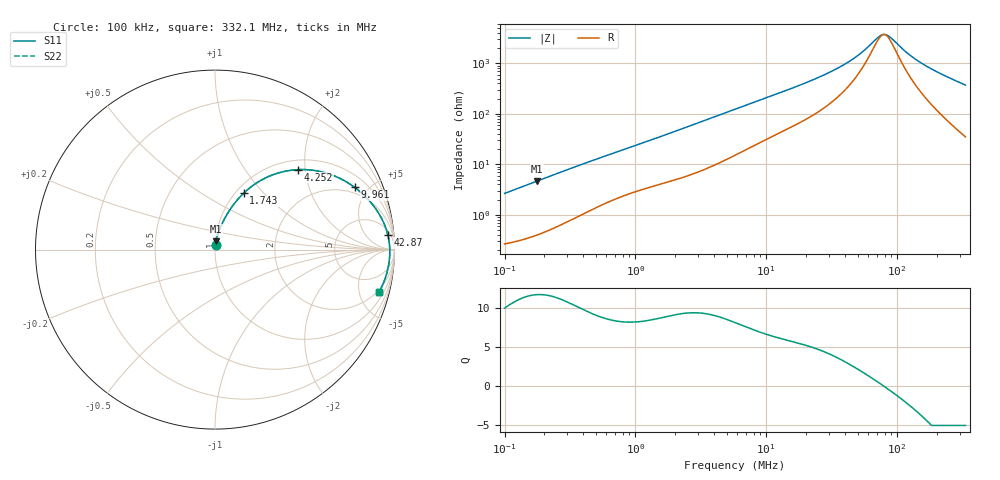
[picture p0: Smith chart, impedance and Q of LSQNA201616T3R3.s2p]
! LSQNA201616T3R3  S-PARAMETER MODEL  ( General Type )
! Model Generated by TAIYO YUDEN Corporation (http://www.ty-top.com)
! Version 2.0
! TAIYO YUDEN Control No. 100810NF25SB-FKC
! Copyright(c) 2007 TAIYO YUDEN CO.,LTD. All Rights Reserved.
! Product Description (link to TY-COMPAS)
! https://ds.yuden.co.jp/TYCOMPAS/or/detail?pn=LSQNA201616T3R3M&u=M
! Products Name : Inductors
! Characteristics :
!  Inductance : 3.3 uH , SRF(min) : 55 MHz , DC Resistance(max) : 0.26 Ohm
!  Rated Current : Saturation :400 mA , Temp Rise : 800 mA (40 degC)
!  Case Size : 2.0 x 1.6 / 0.079 x 0.063 [mm/inch] , Thickness : 1.6 / 0.063 [mm/inch]
!  (Conditions: Temperature = 25 degC , DC Bias Current/Voltage = 0A / 0V)
! External Node Assignments :
!  1  o---GGG---o  2
! GND o---------o GND
! Frequency Range : 0.1MHz  -  332.076389MHz  [ 402 STEP ]
# MHz S RI R 50
! Freq[MHz].  S11 Real  S11 Imag  S21 Real  S21 Imag  S12 Real  S12 Imag  S22 Real  S22 Imag
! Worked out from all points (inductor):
!   401 points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, 100 kHz to 332.1 MHz, reference 50 ohm
!   read as one part in series: L = 4.2 uH near 104.1 kHz
!   highest Q = 11.7 at 176.4 kHz (marker M1), where L = 4.18 uH
!   self-resonance near 79.18 MHz
!   S11 on the Smith chart (normalised r, x): 100 kHz: 1.01, +0.05; 1.743 MHz: 1.09, +0.78; 4.252 MHz: 1.21, +1.83; 9.961 MHz: 1.62, +4.09; 42.87 MHz: 8, +20; 332.1 MHz: 1.70, -7.41
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0.1  0.00334 0.0263  0.9967 -0.0263  0.9967 -0.0263  0.00334 0.0263
0.176395  0.00607 0.0459  0.9939 -0.0459  0.9939 -0.0459  0.00607 0.0459
0.388873  0.0195 0.0963  0.9805 -0.0963  0.9805 -0.0963  0.0195 0.0963
0.840088  0.06 0.1841  0.94 -0.1841  0.94 -0.1841  0.06 0.1841
1.512219  0.1326 0.2862  0.8674 -0.2862  0.8674 -0.2862  0.1326 0.2862
1.742755  0.1603 0.3149  0.8397 -0.3149  0.8397 -0.3149  0.1603 0.3149
2.613956  0.2717 0.3945  0.7283 -0.3945  0.7283 -0.3945  0.2717 0.3945
4.251798  0.4636 0.4456  0.5364 -0.4456  0.5364 -0.4456  0.4636 0.4456
5.762607  0.5922 0.4336  0.4078 -0.4336  0.4078 -0.4336  0.5922 0.4336
9.960991  0.7781 0.3468  0.2219 -0.3468  0.2219 -0.3468  0.7781 0.3468
14.64068  0.8628 0.2689  0.1372 -0.2689  0.1372 -0.2689  0.8628 0.2689
22.4092  0.9213 0.1867  0.0787 -0.1867  0.0787 -0.1867  0.9213 0.1867
32.27618  0.9502 0.1243  0.0498 -0.1243  0.0498 -0.1243  0.9502 0.1243
42.86723  0.9632 0.0814  0.0368 -0.0814  0.0368 -0.0814  0.9632 0.0814
53.57466  0.9693 0.0506  0.0307 -0.0506  0.0307 -0.0506  0.9693 0.0506
74.09842  0.9736 0.00847  0.0264 -0.00847  0.0264 -0.00847  0.9736 0.00847
80.35656  0.9739 -0.00189  0.0261 0.00189  0.0261 0.00189  0.9739 -0.00189
87.14324  0.974 -0.0123  0.026 0.0123  0.026 0.0123  0.974 -0.0123
118.1082  0.972 -0.0525  0.028 0.0525  0.028 0.0525  0.972 -0.0525
150.632  0.9671 -0.0877  0.0329 0.0877  0.0329 0.0877  0.9671 -0.0877
216.9567  0.952 -0.1491  0.048 0.1491  0.048 0.1491  0.952 -0.1491
332.0764  0.9132 -0.2383  0.0868 0.2383  0.0868 0.2383  0.9132 -0.2383
